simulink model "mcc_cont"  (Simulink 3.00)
settings: Solver=ode15s  SolverMode=SingleTasking  StartTime=0.0  StopTime=30  RelTol=1e-3  AbsTol=1e-6

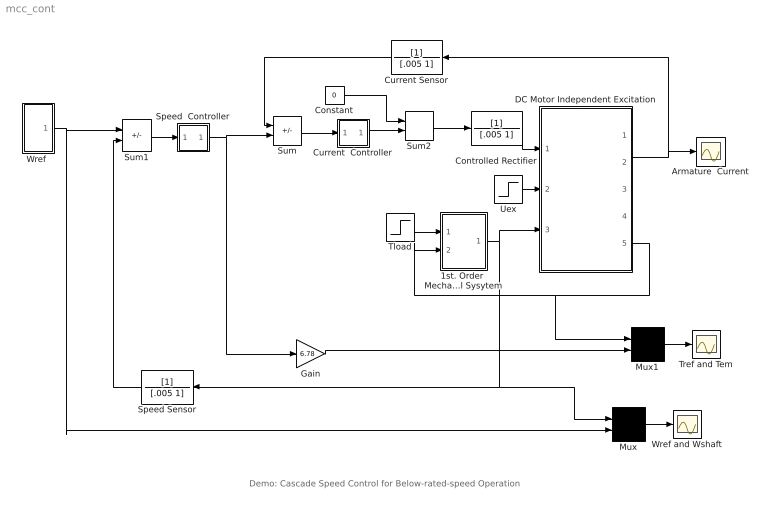
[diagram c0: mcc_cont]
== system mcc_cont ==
  note: Demo: Cascade Speed Control for Below-rated-speed Operation
  1st. Order  Mechanical Sysytem : Subsystem  mask(First Order Mechanical System){J=15, b=.005, wor=0}
      mask prompts: J "Inertia [Kgm]:"; b "Friction Coeficient [Nm seg/rad]:"; wor "Speed Initial Condition [rad/sec]:"
      mask help: This block solves the following differential equation: dW(t)/dt = - W(t)/J + (Tm - Load )/J W(0)=W0
  Armature  Current : Scope
  Constant : Constant  Value=0
  Controlled Rectifier : TransferFcn  Numerator=[1]  Denominator=[.005 1]
  Current  Controller : Subsystem  mask(PI Controller){Kp=.2, Ti=20*.2}
      mask help: G(s)=Kp (Ti s+1)/Ti s
  Current Sensor : TransferFcn  Orientation=left  Numerator=[1]  Denominator=[.005 1]
  DC Motor Independent Excitation : Subsystem  mask(DC Motor ){La=3e-3, Ra=.05, Re=25.2, Ie=[ 0 4.3 5.3 6.2 7.3 8 8.8 10.5], phy=[0 286.5 334.25 382 424 453.62 477.5 525.25], k=.016, ciia=0, f0=0}
      mask prompts: La "Armature Inductance  [Hy]:"; Ra "Armature Resistance [Ohms]:"; Re "Field Resistance  [Ohms]:"; Ie "Field Current Vector [Amp]:"; phy "Field Flux Vector [Wb]:"; k "Motor Constant:"; ciia "Armature Current Initial Condition [Amp]:"; f0 "Flux Initial Condition [Wb]"
  Gain : Gain  Gain=6.78  SaturateOnIntegerOverflow=on
  Mux : Mux  Inputs=2
  Mux1 : Mux  Inputs=2
  Speed  Controller : Subsystem  mask(PI Controller){Kp=40, Ti=15*40}
      mask help: G(s)=Kp (Ti s+1)/Ti s
  Speed Sensor : TransferFcn  Orientation=left  Numerator=[1]  Denominator=[.005 1]
  Sum : Sum  Inputs=-+  SaturateOnIntegerOverflow=on
  Sum1 : Sum  Inputs=+-  SaturateOnIntegerOverflow=on
  Sum2 : Sum  Inputs=++  SaturateOnIntegerOverflow=on
  Tload : Step  Time=25  Before=0  After=2500  SampleTime=0
  Tref and Tem : Scope
  Uex : Step  Time=0  Before=0  After=184  SampleTime=0
  "Wref " : Subsystem  mask(Slope Generator){ti=15, Tr=2, K=60}
      mask prompts: ti "Initial Time [sec]:"; Tr "Rise Time [sec]:"; K "Final Value:"
  Wref and Wshaft : Scope
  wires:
  Uex/1 -> DC Motor Independent Excitation/2(Ve)
  1st. Order  Mechanical Sysytem/1(W) -> DC Motor Independent Excitation/3(Wshaft), Speed Sensor/1, Mux/1
  Mux/1 -> Wref and Wshaft/1
  Tload/1 -> 1st. Order  Mechanical Sysytem/1(Load)
  Sum/1 -> Current  Controller/1(In)
  Current Sensor/1 -> Sum/1
  Sum1/1 -> Speed  Controller/1(In)
  Mux1/1 -> Tref and Tem/1
  Gain/1 -> Mux1/2
  Speed  Controller/1(Out) -> Gain/1, Sum/2
  Speed Sensor/1 -> Sum1/2
  "Wref "/1(slope) -> Sum1/1, Mux/2
  Current  Controller/1(Out) -> Sum2/2
  DC Motor Independent Excitation/5(Tem) -> 1st. Order  Mechanical Sysytem/2(Tm), Mux1/1
  Sum2/1 -> Controlled Rectifier/1
  Controlled Rectifier/1 -> DC Motor Independent Excitation/1(Va)
  DC Motor Independent Excitation/2(Ia) -> Armature  Current/1, Current Sensor/1
  Constant/1 -> Sum2/1

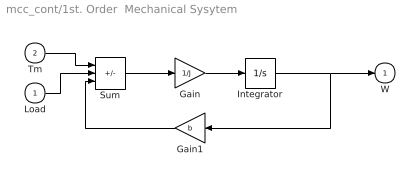
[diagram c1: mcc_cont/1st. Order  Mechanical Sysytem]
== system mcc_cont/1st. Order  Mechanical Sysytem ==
  Load : Inport  Port=1  PortWidth=-1  SampleTime=-1  DataType=auto
  Tm : Inport  Port=2  PortWidth=-1  SampleTime=-1  DataType=auto
  Gain : Gain  Gain=1/J  SaturateOnIntegerOverflow=on
  Gain1 : Gain  Orientation=left  Gain=b  SaturateOnIntegerOverflow=on
  Integrator : Integrator  ExternalReset=none  InitialConditionSource=internal  InitialCondition=wor  LimitOutput=off  UpperSaturationLimit=inf  LowerSaturationLimit=-inf  ShowSaturationPort=off  ShowStatePort=off  AbsoluteTolerance=auto
  Sum : Sum  Inputs=+--  SaturateOnIntegerOverflow=on
  W : Outport  Port=1  InitialOutput=0
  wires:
  Integrator/1 -> W/1, Gain1/1
  Gain1/1 -> Sum/3
  Gain/1 -> Integrator/1
  Sum/1 -> Gain/1
  Tm/1 -> Sum/1
  Load/1 -> Sum/2

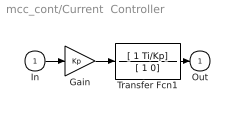
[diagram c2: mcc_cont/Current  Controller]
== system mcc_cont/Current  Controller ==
  In : Inport  Port=1  PortWidth=-1  SampleTime=-1  DataType=auto
  Gain : Gain  Gain=Kp  SaturateOnIntegerOverflow=on
  Transfer Fcn1 : TransferFcn  Numerator=[ 1 Ti/Kp]  Denominator=[ 1 0]
  Out : Outport  Port=1  InitialOutput=0
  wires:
  Transfer Fcn1/1 -> Out/1
  In/1 -> Gain/1
  Gain/1 -> Transfer Fcn1/1

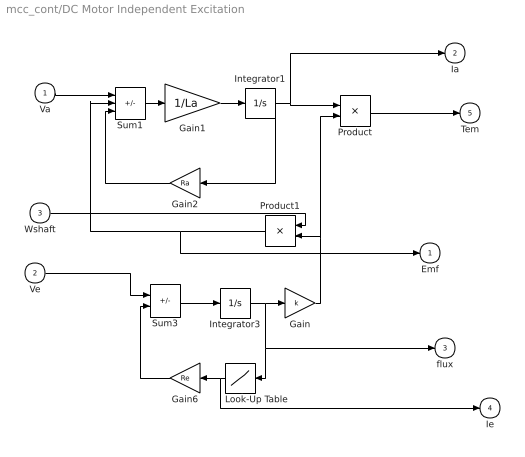
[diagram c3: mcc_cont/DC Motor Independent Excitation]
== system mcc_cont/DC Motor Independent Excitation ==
  Va : Inport  Port=1  PortWidth=-1  SampleTime=-1  DataType=auto
  Ve : Inport  Port=2  PortWidth=-1  SampleTime=-1  DataType=auto
  Wshaft : Inport  Port=3  PortWidth=-1  SampleTime=-1  DataType=auto
  Gain : Gain  Gain=k  SaturateOnIntegerOverflow=on
  Gain1 : Gain  Gain=1/La  SaturateOnIntegerOverflow=on
  Gain2 : Gain  Orientation=left  Gain=Ra  SaturateOnIntegerOverflow=on
  Gain6 : Gain  Orientation=left  Gain=Re  SaturateOnIntegerOverflow=on
  Integrator1 : Integrator  ExternalReset=none  InitialConditionSource=internal  InitialCondition=ciia  LimitOutput=off  UpperSaturationLimit=inf  LowerSaturationLimit=-inf  ShowSaturationPort=off  ShowStatePort=off  AbsoluteTolerance=auto
  Integrator3 : Integrator  ExternalReset=none  InitialConditionSource=internal  InitialCondition=f0  LimitOutput=off  UpperSaturationLimit=inf  LowerSaturationLimit=-inf  ShowSaturationPort=off  ShowStatePort=off  AbsoluteTolerance=auto
  Look-Up Table : Lookup  Orientation=left  InputValues=phy  OutputValues=Ie
  Product : Product  Inputs=2  SaturateOnIntegerOverflow=on
  Product1 : Product  Orientation=left  Inputs=2  SaturateOnIntegerOverflow=on
  Sum1 : Sum  Inputs=+--  SaturateOnIntegerOverflow=on
  Sum3 : Sum  Inputs=+-  SaturateOnIntegerOverflow=on
  Emf : Outport  Port=1  InitialOutput=0
  Ia : Outport  Port=2  InitialOutput=0
  flux : Outport  Port=3  InitialOutput=0
  Ie : Outport  Port=4  InitialOutput=0
  Tem : Outport  Port=5  InitialOutput=0
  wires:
  Look-Up Table/1 -> Gain6/1, Ie/1
  Gain6/1 -> Sum3/2
  Sum1/1 -> Gain1/1
  Gain1/1 -> Integrator1/1
  Gain2/1 -> Sum1/3
  Integrator1/1 -> Gain2/1, Product/1, Ia/1
  Product1/1 -> Sum1/2, Emf/1
  Sum3/1 -> Integrator3/1
  Integrator3/1 -> Gain/1, Look-Up Table/1, flux/1
  Gain/1 -> Product/2, Product1/2
  Product/1 -> Tem/1
  Va/1 -> Sum1/1
  Wshaft/1 -> Product1/1
  Ve/1 -> Sum3/1

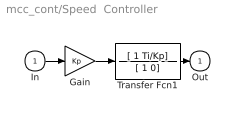
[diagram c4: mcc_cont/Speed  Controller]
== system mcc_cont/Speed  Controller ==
  In : Inport  Port=1  PortWidth=-1  SampleTime=-1  DataType=auto
  Gain : Gain  Gain=Kp  SaturateOnIntegerOverflow=on
  Transfer Fcn1 : TransferFcn  Numerator=[ 1 Ti/Kp]  Denominator=[ 1 0]
  Out : Outport  Port=1  InitialOutput=0
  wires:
  Gain/1 -> Transfer Fcn1/1
  In/1 -> Gain/1
  Transfer Fcn1/1 -> Out/1

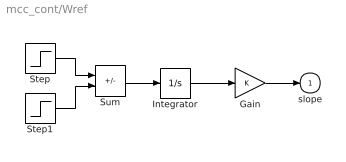
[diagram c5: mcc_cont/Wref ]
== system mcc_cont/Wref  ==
  Gain : Gain  Gain=K  SaturateOnIntegerOverflow=on
  Integrator : Integrator  ExternalReset=none  InitialConditionSource=internal  InitialCondition=0  LimitOutput=off  UpperSaturationLimit=inf  LowerSaturationLimit=-inf  ShowSaturationPort=off  ShowStatePort=off  AbsoluteTolerance=auto
  Step : Step  Time=ti  Before=0  After=1/Tr  SampleTime=0
  Step1 : Step  Time=ti+Tr  Before=0  After=1/Tr  SampleTime=0
  Sum : Sum  Inputs=+-  SaturateOnIntegerOverflow=on
  slope : Outport  Port=1  InitialOutput=0
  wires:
  Integrator/1 -> Gain/1
  Gain/1 -> slope/1
  Sum/1 -> Integrator/1
  Step/1 -> Sum/1
  Step1/1 -> Sum/2
